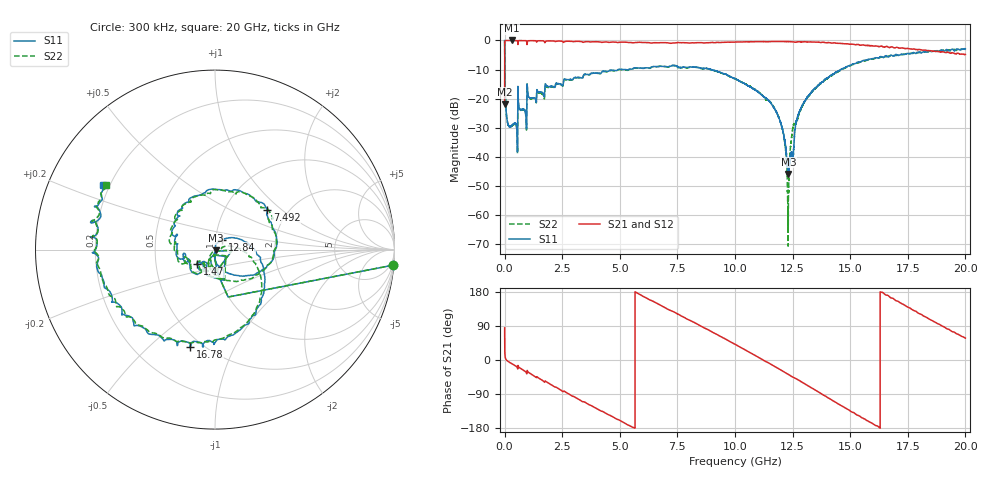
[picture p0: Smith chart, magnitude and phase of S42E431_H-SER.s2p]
! Created Wed Nov 25 22:16:51 2020
# khz S ma R 50
! 2 Port Network Data from SP1.SP block
! freq  magS11  angS11  magS21  angS21  magS12  angS12  magS22  angS22
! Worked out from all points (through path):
!   20001 points, 300 kHz to 20 GHz, reference 50 ohm
!   highest |S21| = -0.01 dB at 302.3 MHz (marker M1); lowest = -22.0 dB at 300 kHz (marker M2)
!   group delay of S21, straight-line fit = 92.5 ps
!   lowest |S11| = -45.9 dB at 12.31 GHz (marker M3), VSWR 1.01, Z = 50.4 - j0.319 ohm
!   |S11| at or under -10 dB: 11.38 MHz to 4.927 GHz (4.916 GHz wide, 199 % of centre); 5.191 GHz to 5.383 GHz (192.4 MHz wide, 3.64 % of centre); 8.962 GHz to 14.59 GHz (5.63 GHz wide, 47.8 % of centre)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
!   |S22| runs from -70.7 to 0.0 dB; largest |S21 - S12| = 0.016
!   S11 on the Smith chart (normalised r, x): 300 kHz: 2, -23; 1.47 GHz: 0.81, -0.13; 7.492 GHz: 1.58, +0.80; 12.84 GHz: 1.08, +0.11; 16.78 GHz: 0.43, -0.68; 20 GHz: 0.18, +0.26
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300  0.9941 -5.0  0.07947 84.7  0.07922 84.7  0.9956 -5.0
126300  0.03909 -92.6  0.9979 -2.5  0.999 -2.5  0.03896 -92.4
302300  0.03436 -99.4  0.9993 -9.4  0.998 -9.4  0.03369 -98.7
1470300  0.1278 -140.8  0.9861 -47.3  0.9863 -47.3  0.1266 -134.5
3334300  0.2268 158.0  0.9556 -108.3  0.956 -108.2  0.2238 168.9
5158300  0.3167 108.2  0.9351 -164.7  0.9339 -164.6  0.3133 104.4
6667300  0.3568 61.3  0.9108 147.9  0.9103 147.8  0.3561 57.0
7492300  0.3654 36.9  0.9154 121.9  0.9122 122.0  0.3666 27.8
8905300  0.3207 -12.5  0.9162 77.4  0.9191 77.3  0.3184 -13.1
1.00003e7  0.2216 -41.9  0.9374 41.6  0.936 41.6  0.2207 -52.8
1.17353e7  0.06503 -87.3  0.9579 -17.5  0.9579 -17.5  0.06552 -121.7
1.20753e7  0.02875 -94.4  0.9575 -29.5  0.9577 -29.4  0.0279 -133.7
1.22413e7  0.009747 -82.2  0.9573 -35.6  0.9546 -35.6  0.007622 -134.7
1.23143e7  0.005047 -38.8  0.9561 -38.0  0.9564 -38.0  0.0009309 -7.6
1.25053e7  0.01007 41.0  0.9458 -45.0  0.9445 -45.1  0.03086 22.0
1.28433e7  0.06621 53.4  0.9465 -56.1  0.9451 -56.0  0.06352 18.5
1.33343e7  0.1299 29.2  0.9407 -74.0  0.9399 -74.1  0.1303 3.0
1.50473e7  0.3823 -47.5  0.8638 -136.4  0.8672 -136.1  0.3746 -47.9
1.66673e7  0.5229 -101.2  0.761 169.0  0.7647 168.3  0.5365 -104.0
1.67813e7  0.5607 -104.3  0.7755 163.7  0.7723 164.5  0.5388 -107.5
1.82733e7  0.6326 -154.6  0.6817 113.6  0.672 113.9  0.6399 -156.7
2e7  0.7185 149.8  0.5736 57.6  0.5746 58.0  0.7091 149.0
